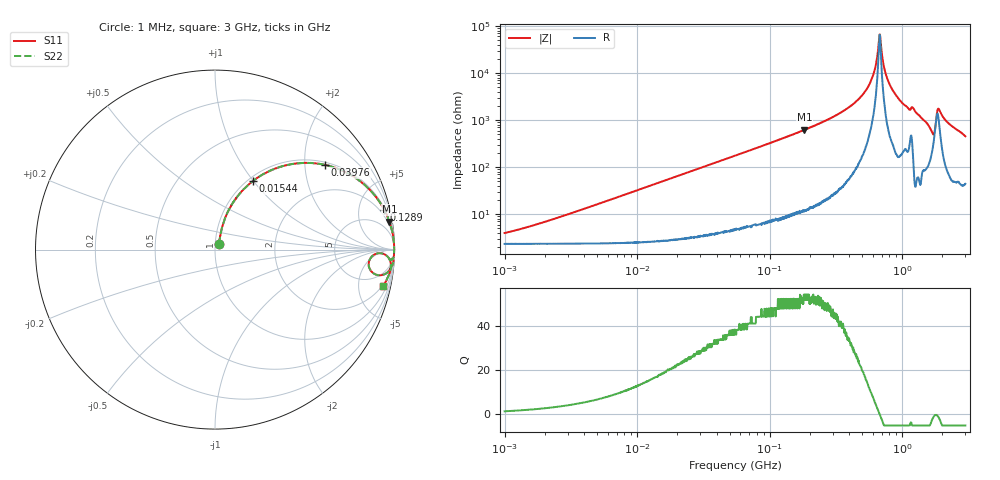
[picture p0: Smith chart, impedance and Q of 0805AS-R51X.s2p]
!s-Parameter Generated by FASTRON Sdn. Bhd.
!FASTRON P/N : 0805AS-R51X
!Keysight Technologies: E4991B_MY54100416_A.01.15
!Date: Mon Jun 15 12:55:16 2026
!Version  :Rev01  Mon Jun 15 12:55:16 2026
!Data & Calibration Information:
!Freq  S11  S21  S12  S22
!PortZ  Port1:50+j0  Port2:50+j0
!When reading reference impedance value at option line is always used.
! Remarks : This data is being provided solely for informational purposes.
# Hz S dB R 50
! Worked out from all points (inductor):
!   1601 points, 1 MHz to 3 GHz, reference 50 ohm
!   read as one part in series: L = 512 nH near 2.205 MHz
!   highest Q = 54 at 182.9 MHz (marker M1), where L = 540 nH
!   self-resonance near 675.3 MHz
!   S11 on the Smith chart (normalised r, x): 1 MHz: 1.05, +0.06; 15.44 MHz: 1.05, +0.99; 39.76 MHz: 1.08, +2.54; 128.9 MHz: 1.17, +8.42; 3 GHz: 1.89, -9.04
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1000000  -28.20 52.2  -0.20 -1.8  -0.20 -1.8  -28.20 52.2
3804036  -18.40 72.2  -0.27 -6.8  -0.27 -6.8  -18.40 72.2
1.447069e7  -7.68 62.4  -1.04 -24.3  -1.04 -24.3  -7.68 62.4
1.544333e7  -7.22 61.1  -1.14 -25.8  -1.14 -25.8  -7.22 61.1
3.976269e7  -2.22 37.5  -4.31 -50.8  -4.31 -50.8  -2.22 37.5
5.504702e7  -1.31 29.2  -6.23 -59.3  -6.23 -59.3  -1.31 29.2
1.288778e8  -0.28 13.3  -12.80 -75.6  -12.80 -75.6  -0.28 13.3
1.829372e8  -0.14 9.1  -16.00 -79.8  -16.00 -79.8  -0.14 9.1
2.083556e8  -0.10 7.9  -17.30 -81.0  -17.30 -81.0  -0.10 7.9
3.631036e8  -0.03 3.6  -24.00 -84.9  -24.00 -84.9  -0.03 3.6
5.001674e8  -0.02 1.7  -30.60 -85.4  -30.60 -85.4  -0.02 1.7
5.988949e8  -0.01 0.7  -38.50 -82.1  -38.50 -82.1  -0.01 0.7
6.753166e8  -0.01 0.0  -56.40 -9.5  -56.40 -9.5  -0.01 0.0
6.958997e8  -0.01 -0.2  -50.30 60.6  -50.30 60.6  -0.01 -0.2
7.42674e8  -0.01 -0.5  -40.70 80.8  -40.70 80.8  -0.01 -0.5
7.925923e8  -0.01 -0.9  -36.00 84.1  -36.00 84.1  -0.01 -0.9
9.878038e8  -0.04 -2.4  -27.70 83.2  -27.70 83.2  -0.04 -2.4
1.218836e9  -0.04 -3.3  -24.90 83.3  -24.90 83.3  -0.04 -3.3
1.67892e9  -0.66 -8.9  -15.60 59.4  -15.60 59.4  -0.66 -8.9
1.902655e9  -0.26 -2.9  -24.70 58.3  -24.70 58.3  -0.26 -2.9
2.221924e9  -0.14 -6.5  -19.00 78.7  -19.00 78.7  -0.14 -6.5
3e9  -0.38 -12.1  -13.50 72.3  -13.50 72.3  -0.38 -12.1
